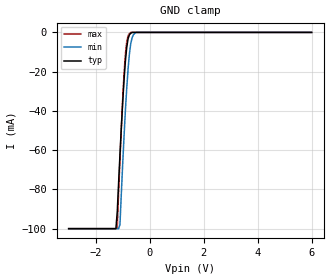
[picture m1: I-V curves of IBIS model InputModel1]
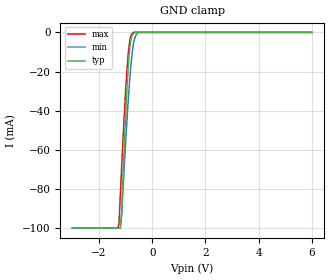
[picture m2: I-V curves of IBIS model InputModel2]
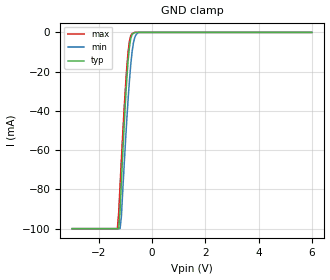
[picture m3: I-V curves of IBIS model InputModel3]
[IBIS Ver]   2.1
[File name]   e_800cel.ibs   | e_= TSOP, f800ce= abbr chip name,
|   | l = 2.7 to 3.3V Vcc
[File Rev]   2.00
[Date]   2-April-1996
[Source]   File generated from lab measurements at Intel Corporation
[Notes]   Rev 2.00 All data was replaced by actual measurements
   performed in a lab.
[Disclaimer] INTEL DEVELOPER'S SOFTWARE LICENSE AGREEMENT
| BY USING THIS SOFTWARE, YOU ARE AGREEING TO BE BOUND
| BY THE TERMS OF THIS AGREEMENT.  DO NOT USE THE SOFTWARE
| UNTIL YOU HAVE CAREFULLY READ AND AGREED TO THE FOLLOWING
| TERMS AND CONDITIONS.  IF YOU DO NOT AGREE TO THE TERMS
| OF THIS AGREEMENT, PROMPTLY RETURN THE SOFTWARE PACKAGE
| AND ANY ACCOMPANYING ITEMS.
| IF YOU USE THIS SOFTWARE, YOU WILL BE BOUND BY THE TERMS
| OF THIS AGREEMENT
| LICENSE: Intel Corporation ("Intel") grants you the non-exclusive right
| to use the enclosed software program ("Software").  You will not use,
| copy, modify, rent, sell or transfer the Software or any portion
| thereof, except as provided in this Agreement.
| System OEM Developers may:
| 1.   Copy the Software for support, backup or archival purposes;
| 2.   Install, use, or distribute Intel owned Software in object code
|   only;
| 3.   Modify and/or use Software source code that Intel directly makes
|   available to you as an OEM Developer;
| 4.   Install, use, modify, distribute, and/or make or have made
|   derivatives ("Derivatives") of Intel owned Software under the
|   terms and conditions in this Agreement, ONLY if you are a System
|   OEM Developer and NOT an end-user.
| RESTRICTIONS:
| YOU WILL NOT:
| 1.   Copy the Software, in whole or in part, except as provided for
|   in this Agreement;
| 2.   Decompile or reverse engineer any Software provided in object
|   code format;
| 3.   Distribute any Software or Derivative code to any end-users,
|   unless approved by Intel in a prior writing.
| TRANSFER: You may transfer the Software to another OEM
| Developer if the receiving party agrees to the terms of this
| Agreement at the sole risk of any receiving party.
| OWNERSHIP AND COPYRIGHT OF SOFTWARE:
| Title to the Software and all copies thereof remain with Intel
| or its vendors.  The Software is copyrighted and is protected by
| United States and international copyright laws.  You will not
| remove the copyright notice from the Software.  You agree to
| prevent any unauthorized copying of the Software.
| DERIVATIVE WORK: OEM Developers that make or have made
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[Copyright]   Copyright 1996, Intel Corporation, All Rights Reserved
[Component]   E28F800CE   | 48-lead TSOP package, 28F800CE
[Manufacturer]  Intel   | Boot Block (tm)
|   | operating in 2.7-3.3V Vcc range
[Package]
|Variable   typ   min   max
|The following values apply for the leadframe.
R_pkg   135m   126m   144m
L_pkg   3.95nH   3.62nH   4.28nH
C_pkg   0.39pF   0.38pF   0.40pF
|*****************************Pin Definitions**********************************
[Pin]   signal_name   model_name   R_pin   L_pin   C_pin
 1   A15   InputModel3
 2   A14   InputModel3
 3   A13   InputModel3
 4   A12   InputModel3
 5   A11   InputModel3
 6   A10   InputModel3
 7   A09   InputModel3
 8   A08   InputModel3
 9   NC   InputModel4
10   NC   InputModel4
11   WE#   InputModel1
12   RP#   InputModel1
13   VPP   POWER
14   WP#   InputModel1
15   NC   InputModel4
16   A18   InputModel3
17   A17   InputModel3
18   A07   InputModel3
19   A06   InputModel3
20   A05   InputModel3
21   A04   InputModel3
22   A03   InputModel3
23   A02   InputModel3
24   A01   InputModel3
25   A00   InputModel2
26   CE#   InputModel1
27   GND   GND
28   OE#   InputModel1
29   DQ0   InputOutput
30   DQ8   InputOutput
31   DQ1   InputOutput
32   DQ9   InputOutput
33   DQ2   InputOutput
34   DQ10   InputOutput
35   DQ3   InputOutput
36   DQ11   InputModel3
37   VCC   POWER
38   DQ4   InputModel4
39   DQ12   InputOutput
40   DQ5   InputModel3
41   DQ13   InputOutput
42   DQ6   InputOutput
43   DQ14   InputOutput
44   DQ7   InputOutput
45   DQ15   InputOutput
46   GND   GND
47   BYTE#   InputModel2
48   A16   InputModel2
|***********************Input Model 4******************************
[Model]   InputModel4
Model_type   Input
|   Model for NC pins (Numbers 9, 10 & 15).
Vinl = 0.8V
Vinh = 2.0V
|Variable   Typ   Min   Max
C_comp   5.61p   NA   7.6p
[Voltage Range]   3.0V   2.7V   3.3V
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| Models and submodels in the file (5): InputModel1 (Input), InputModel2 (Input), InputModel3 (Input), InputModel4 (Input), InputOutput (I/O)
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|*********************Input Model 1************************************
[Model]   InputModel1
Model_type   Input
|   Model for WE#, WP#, RP#, OE# & CE#.
Vinl = 0.8V
Vinh = 2.0V
|Variable   Typ   Min   Max
C_comp   5.61p   NA   7.6p
[Voltage Range]   3.0V   2.7V   3.3V
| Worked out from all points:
|   GND clamp passes 1 mA (typ) near -0.74 V on its own axis
[GND_clamp]
|Voltage  I(typ)   I(min)   I(max)
-3V       -100mA     -100mA     -100mA
-1.25V    -100mA     -100mA     -100mA
-1.2V     -91.38mA   -100mA     -99.69mA
-1.1V     -62.33mA   -97.89mA   -64.9mA
-1V       -35.99mA   -67.36mA   -34.11mA
-900mV    -14.83mA   -40.08mA   -11.26mA
-850mV    -7.774mA   -28.73mA   -4.823mA
-800mV    -3.283mA   -18.71mA   -1.668mA
-700mV    -471.4uA   -5.736mA   0A
-600mV    0A         -1.158mA   0A
-500mV    0A         0A         0A
6V        0A         0A         0A
[Power_clamp]
| Input buffer circuits of this product do not intrinsically
| require a [Power_clamp] definition.  This zero current
| [Power_clamp] table is provided for the compatibility with
| some IBIS parsers.
|Voltage  I(typ)   I(min)   I(max)
-3V       0A         0A         0A
0V        0A         0A         0A
3V        0A         0A         0A
6V        0A         0A         0A
|*********************Input Model 2******************************
[Model]   InputModel2
Model_type   Input
|   Model for A[0], A[16] & BYTE# pins.
Vinl = 0.8V
Vinh = 2.0V
|Variable   Typ   Min   Max
C_comp   5.61p   NA   7.6p
[Voltage Range]   3.0V   2.7V   3.3V
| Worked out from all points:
|   GND clamp passes 1 mA (typ) near -0.73 V on its own axis
[GND_clamp]
|Voltage  I(typ)   I(min)   I(max)
-3V       -100mA     -100mA     -100mA
-1.3V     -100mA     -100mA     -100mA
-1.25V    -100mA     -100mA     -97.92mA
-1.2V     -100mA     -100mA     -83.24mA
-1.15V    -91.8mA    -93.8mA    -68.92mA
-1V       -42.09mA   -56.51mA   -29.98mA
-900mV    -16.78mA   -34.42mA   -10.53mA
-850mV    -8.519mA   -25.07mA   -4.731mA
-800mV    -3.472mA   -16.7mA    -1.714mA
-700mV    -480.5uA   -5.462mA   0A
-500mV    0A         0A         0A
6V        0A         0A         0A
[Power_clamp]
| Input buffer circuits of this product do not intrinsically
| require a [Power_clamp] definition.  This zero current
| [Power_clamp] table is provided for the compatibility with
| some IBIS parsers.
|Voltage  I(typ)   I(min)   I(max)
-3V       0A         0A         0A
0V        0A         0A         0A
3V        0A         0A         0A
6V        0A         0A         0A
|***********************Input Model 3******************************
[Model]   InputModel3
Model_type   Input
|   Model for A[15:1] & A[17:18].
Vinl = 0.8V
Vinh = 2.0V
|Variable   Typ   Min   Max
C_comp   5.61p   NA   7.6p
[Voltage Range]   3.0V   2.7V   3.3V
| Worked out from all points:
|   GND clamp passes 1 mA (typ) near -0.74 V on its own axis
[GND_clamp]
|Voltage  I(typ)   I(min)   I(max)
-3V       -100mA     -100mA     -100mA
-1.3V     -100mA     -100mA     -100mA
-1.25V    -100mA     -100mA     -91.69mA
-1.2V     -90.85mA   -100mA     -78.06mA
-1.15V    -76.19mA   -93.92mA   -64.74mA
-1.05V    -48.54mA   -68.57mA   -39.73mA
-950mV    -24.46mA   -45.15mA   -18.47mA
-850mV    -7.709mA   -25.05mA   -4.698mA
-750mV    -1.198mA   -10.09mA   -626uA
-650mV    0A         -2.645mA   0A
-500mV    0A         0A         0A
6V        0A         0A         0A
[Power_clamp]
| Input buffer circuits of this product do not intrinsically
| require a [Power_clamp] definition.  This zero current
| [Power_clamp] table is provided for the compatibility with
| some IBIS parsers.
|Voltage  I(typ)   I(min)   I(max)
-3V       0A         0A         0A
0V        0A         0A         0A
3V        0A         0A         0A
6V        0A         0A         0A
